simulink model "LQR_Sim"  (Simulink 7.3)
settings: Solver=ode45  StartTime=0.0  StopTime=20  RelTol=1e-3
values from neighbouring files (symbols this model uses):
  r2d = 180/pi    (= 57.2957795131)    [LQR_Design.m]    (also in init.m; pl.m)
undefined symbols (not defined in the file or in its folder): Avl, Avp, Bvl, Bvp, Cvl, Cvp, Dvl, Dvp, Kpr, Kq

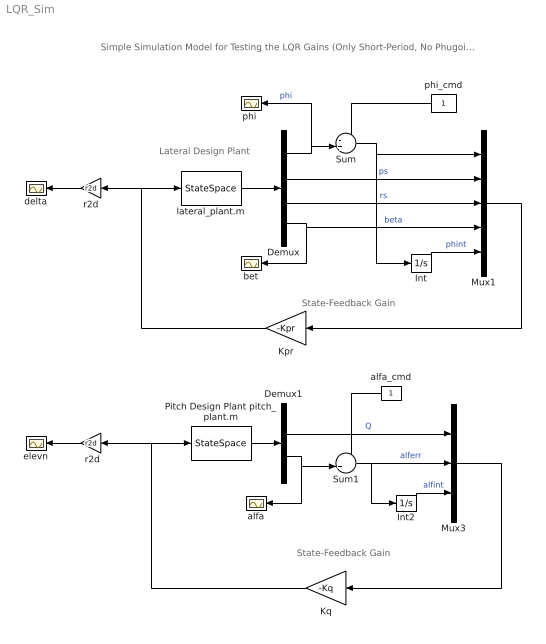
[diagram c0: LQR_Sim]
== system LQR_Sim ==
  note: Simple Simulation Model for Testing the LQR Gains (Only Short-Period, No Phugoid)
  note: Lateral Design Plant
  note: State-Feedback Gain
  note: State-Feedback Gain
  " r2d" : Gain  Gain=r2d  ParameterDataType=fixdt(1, 16)  ParameterScaling=2^0  OutDataType=fixdt(1, 16)  OutScaling=2^0
  Demux : Demux
  Demux1 : Demux  Outputs=2
  Int : Integrator
  Int2 : Integrator
  Kpr : Gain  Gain=-Kpr  Multiplication=Matrix(K*u)  ParameterDataType=fixdt(1, 16)  ParameterScaling=2^0  OutDataType=fixdt(1, 16)  OutScaling=2^0
  Kq : Gain  Gain=-Kq  Multiplication=Matrix(K*u)  ParameterDataType=fixdt(1, 16)  ParameterScaling=2^0  OutDataType=fixdt(1, 16)  OutScaling=2^0
  Mux1 : Mux  Inputs=5
  Mux3 : Mux  Inputs=3
  Pitch Design Plant pitch_plant.m : StateSpace  A=Avp  B=Bvp  C=Cvp  D=Dvp
  Sum : Sum  Inputs=-+|  OutDataType=fixdt(1, 16)  OutScaling=2^0
  Sum1 : Sum  Inputs=-+|  OutDataType=fixdt(1, 16)  OutScaling=2^0
  alfa : Scope
  alfa_cmd : Constant  OutDataType=fixdt(1, 16)  OutScaling=2^0
  bet : Scope
  delta : Scope
  elevn : Scope
  lateral_plant.m : StateSpace  A=Avl  B=Bvl  C=Cvl  D=Dvl
  "phi " : Scope
  phi_cmd : Constant  OutDataType=fixdt(1, 16)  OutScaling=2^0
  r2d : Gain  Gain=r2d  ParameterDataType=fixdt(1, 16)  ParameterScaling=2^0  OutDataType=fixdt(1, 16)  OutScaling=2^0
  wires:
  Kpr/1 -> lateral_plant.m/1, r2d/1
  lateral_plant.m/1 -> Demux/1
  Demux/2 -> Mux1/2  "ps"
  Demux/3 -> Mux1/3  "rs"
  Demux/4 -> Mux1/4, bet/1  "beta"
  Int/1 -> Mux1/5  "phint"
  Demux/1 -> Sum/2, "phi "/1  "phi"
  Sum/1 -> Mux1/1, Int/1
  phi_cmd/1 -> Sum/1
  Mux1/1 -> Kpr/1
  r2d/1 -> delta/1
  Pitch Design Plant pitch_plant.m/1 -> Demux1/1
  Kq/1 -> Pitch Design Plant pitch_plant.m/1, " r2d"/1
  " r2d"/1 -> elevn/1
  Mux3/1 -> Kq/1
  Demux1/1 -> Mux3/1  "Q"
  Int2/1 -> Mux3/3  "alfint"
  Demux1/2 -> Sum1/2, alfa/1
  Sum1/1 -> Mux3/2, Int2/1  "alferr"
  alfa_cmd/1 -> Sum1/1
